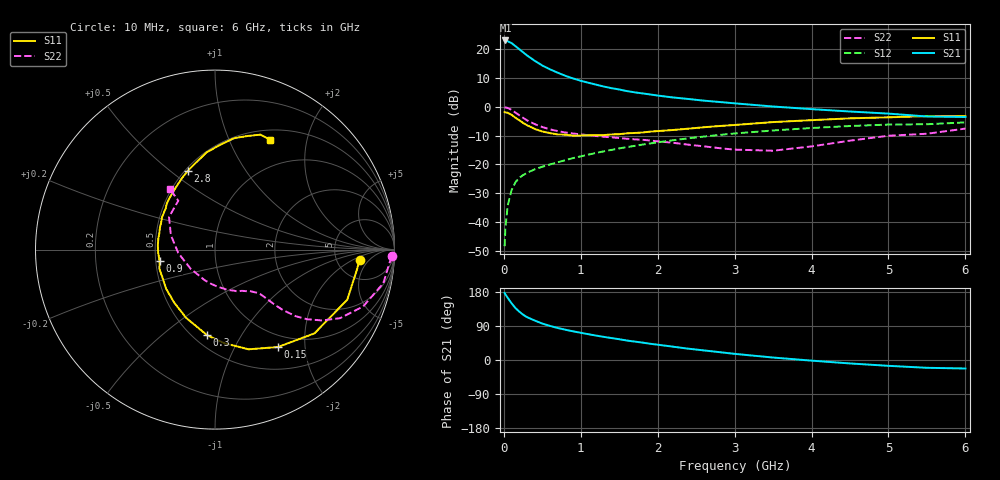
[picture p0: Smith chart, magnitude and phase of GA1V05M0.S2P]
! Infineon Technologies  Discrete & RF Semiconductors
! BF775
! Si NPN RF Bipolar Junction Transistor in SOT23
! VCE = 1 V  IC = 5 mA
! Common Emitter S-Parameters:  May  1996
# GHz  S  MA  R  50
!  f  S11  S21  S12  S22
! GHz  MAG  ANG  MAG  ANG  MAG  ANG  MAG  ANG
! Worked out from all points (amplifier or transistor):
!   36 points, 10 MHz to 6 GHz, reference 50 ohm
!   highest |S21| = 23.0 dB at 20 MHz (marker M1)
!   |S21| within 3 dB of that: start of sweep to 199 MHz
!   unconditionally stable (mu >= 1): 705.1 MHz to end of sweep
!   at 250 MHz: K = 0.51, MSG = 21.3 dB, |S12| = -23.7 dB
!   at 1.4 GHz: K = 1.17, MAG = 8.2 dB, |S12| = -15.0 dB
!   at 6 GHz: K = 1.03, MAG = -0.2 dB, |S12| = -5.4 dB
!   S11 on the Smith chart (normalised r, x): 10 MHz: 8.36, -2.91; 150 MHz: 0.81, -1.52; 300 MHz: 0.59, -0.72; 900 MHz: 0.52, -0.07; 2.8 GHz: 0.52, +0.58; 6 GHz: 0.62, +1.43
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0.01  0.8074 -4.3  14.19 177.0  0.0038 87.6  0.9852 -2.2
0.02  0.7973 -8.7  14.2 173.4  0.0077 84.7  0.9741 -4.6
0.05  0.7878 -20.8  13.77 164.1  0.0192 79.5  0.9564 -11.3
0.1  0.7246 -40.1  12.77 149.8  0.0357 70.2  0.8842 -21.0
0.15  0.6463 -57.1  11.34 137.2  0.0488 62.7  0.7951 -28.7
0.2  0.5862 -71.4  10.03 127.8  0.0585 58.3  0.7153 -33.5
0.25  0.5239 -84.4  8.854 119.6  0.0652 54.6  0.6432 -37.1
0.3  0.4792 -95.2  7.833 113.2  0.0713 53.1  0.5835 -39.5
0.4  0.4133 -112.8  6.307 104.2  0.082 51.3  0.5018 -41.8
0.5  0.3729 -127.5  5.212 96.2  0.091 50.9  0.4455 -42.8
0.6  0.349 -141.2  4.476 89.9  0.0998 51.7  0.4058 -43.4
0.7  0.3315 -151.8  3.912 84.5  0.1088 52.1  0.3787 -43.9
0.9  0.315 -168.5  3.107 75.7  0.1286 52.5  0.3439 -45.1
1.1  0.3193 175.4  2.614 68.0  0.1478 52.8  0.321 -47.5
1.3  0.3228 164.0  2.248 61.0  0.1685 52.4  0.3018 -50.1
1.6  0.3462 148.5  1.876 51.4  0.1998 51.1  0.2786 -55.7
2.2  0.3956 126.7  1.452 35.1  0.2627 46.0  0.2373 -71.7
2.8  0.4635 109.2  1.214 20.8  0.3245 39.3  0.1916 -96.7
3.5  0.5429 95.1  1.012 6.5  0.3882 30.1  0.1727 -142.1
4.5  0.6306 80.1  0.828 -9.1  0.4641 16.8  0.2584 162.0
5.5  0.689 68.4  0.679 -20.6  0.4981 2.9  0.3406 126.9
6  0.6842 63.4  0.665 -22.4  0.5363 -0.9  0.4187 126.7
